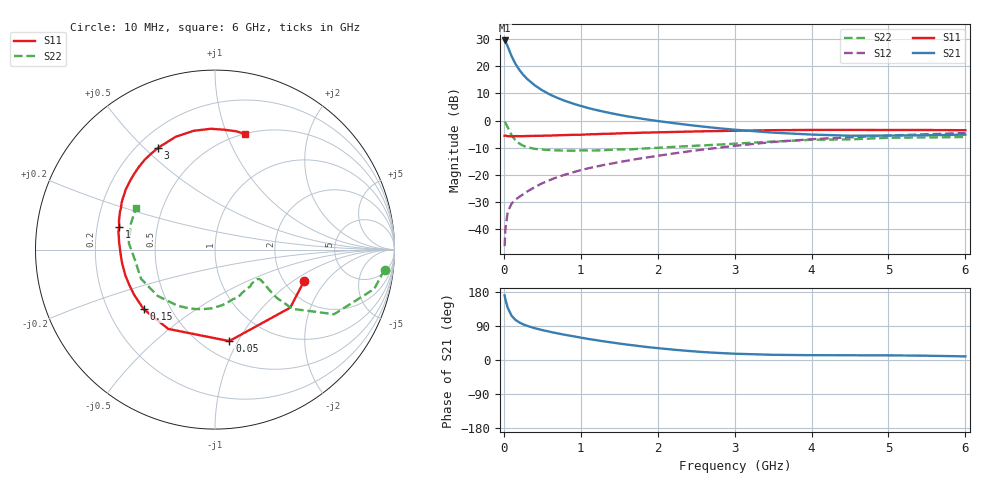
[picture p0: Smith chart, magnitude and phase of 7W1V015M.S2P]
! Infineon Technologies  Discrete & RF Semiconductors
! BFS17W
! Si NPN RF Bipolar Junction Transistor in SOT323
! VCE = 1 V  IC = 15 mA
! Common Emitter S-Parameters:  August  1999
# GHz  S  MA  R  50
!  f  S11  S21  S12  S22
! GHz  MAG  ANG  MAG  ANG  MAG  ANG  MAG  ANG
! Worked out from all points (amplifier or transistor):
!   36 points, 10 MHz to 6 GHz, reference 50 ohm
!   highest |S21| = 29.5 dB at 10 MHz (marker M1)
!   |S21| within 3 dB of that: start of sweep to 61.19 MHz
!   unconditionally stable (mu >= 1): 235.6 MHz to end of sweep
!   at 250 MHz: K = 1.04, MAG = 20.9 dB, |S12| = -27.2 dB
!   at 1.4 GHz: K = 1.35, MAG = 5.7 dB, |S12| = -15.8 dB
!   at 6 GHz: K = 1.12, MAG = -2.4 dB, |S12| = -4.6 dB
!   S11 on the Smith chart (normalised r, x): 10 MHz: 2.56, -1.23; 50 MHz: 0.66, -0.92; 150 MHz: 0.35, -0.32; 1 GHz: 0.30, +0.11; 3 GHz: 0.28, +0.55; 6 GHz: 0.51, +1.17
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0.01  0.5267 -19.2  29.72 170.5  0.0049 80.5  0.9515 -6.7
0.02  0.5295 -37.6  28.65 160.5  0.01 75.5  0.9135 -13.9
0.05  0.5159 -81.1  23.03 137.8  0.0209 62.3  0.7547 -28.5
0.1  0.5128 -120.5  15.38 117.0  0.0296 52.3  0.5432 -37.4
0.15  0.5177 -140.1  11.1 106.0  0.0351 50.5  0.434 -38.0
0.2  0.5163 -150.9  8.613 99.3  0.0394 53.0  0.379 -36.7
0.25  0.5168 -158.4  6.997 94.3  0.0439 54.3  0.3445 -35.2
0.3  0.5195 -163.6  5.888 90.4  0.0492 56.5  0.3257 -34.4
0.4  0.5231 -171.4  4.466 84.0  0.0594 59.5  0.302 -33.5
0.5  0.5257 -176.5  3.597 79.0  0.0704 61.7  0.2937 -33.8
0.6  0.5298 179.3  3.006 74.4  0.0808 63.1  0.287 -35.2
0.8  0.5406 172.3  2.289 66.3  0.1016 64.0  0.2802 -40.3
1  0.5483 166.5  1.859 59.1  0.1229 64.3  0.2836 -45.9
1.1  0.5581 163.5  1.697 55.5  0.1326 64.2  0.282 -50.0
1.3  0.5703 158.1  1.455 49.2  0.1526 63.7  0.2844 -57.9
1.6  0.5875 151.0  1.2 40.7  0.1824 63.2  0.2936 -69.6
2.2  0.6167 137.2  0.9 27.4  0.2475 61.1  0.3279 -93.6
3  0.6497 119.3  0.679 16.6  0.343 54.8  0.3754 -123.5
3.5  0.6657 109.2  0.6 13.7  0.4036 49.3  0.4109 -141.1
4.5  0.6737 92.0  0.526 12.5  0.4909 36.4  0.4503 -173.0
5.5  0.6698 79.9  0.536 11.3  0.5603 25.4  0.4907 162.9
6  0.665 75.2  0.552 9.5  0.5885 20.0  0.4976 152.3
